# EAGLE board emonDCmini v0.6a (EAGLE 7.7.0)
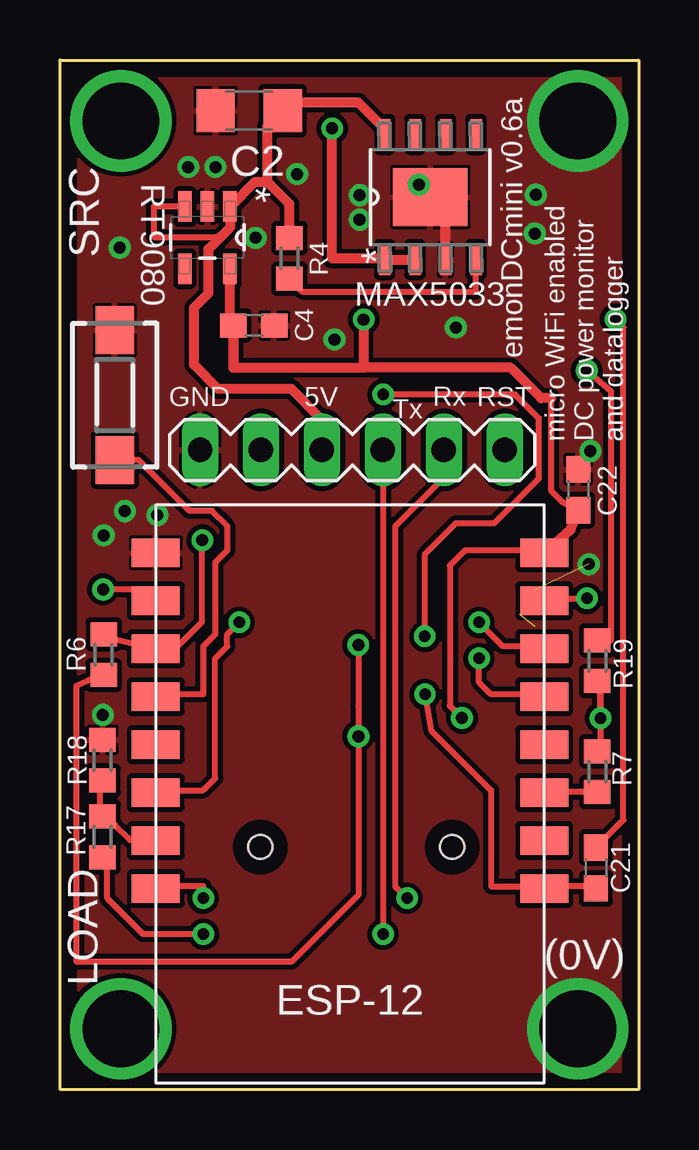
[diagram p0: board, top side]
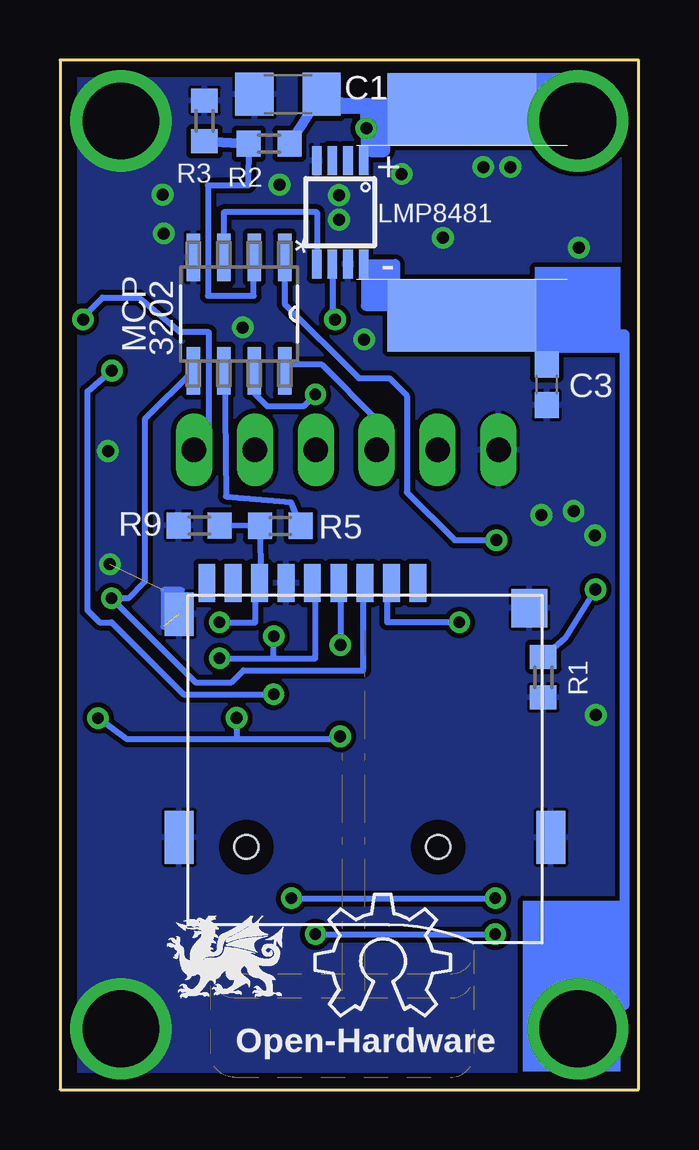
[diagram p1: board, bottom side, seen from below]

Size 24.13 x 42.93 mm. Coordinates in mm from the lower left corner, seen from the top.
Outline: 0,42.93 24.13,42.93 24.13,0 0,0 0,42.93
Copper layers (1*16): Top 0.035mm / dielectric 1.5mm / Bottom 0.035mm
Design rules "default *": minimum track width 10mil, minimum drill 19mil, track to track 8mil, track to pad 8mil, pad to pad 8mil, via to via 8mil, smd to smd 8mil, copper to edge 25mil, drill to drill 8mil, minimum pad ring 10mil, minimum via ring 8mil, stop-mask expansion 4mil, vias tented up to drill 0mil, thermal gap 5mil
Net classes: 1 power: width 1.016 mm; 2 thin_power: width 0.254 mm

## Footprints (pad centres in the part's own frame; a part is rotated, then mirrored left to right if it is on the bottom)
C1206 = smd 1.6 x 1.8: 1 -1.4,0; 2 1.4,0
C0603 = smd 1.1 x 1: 1 -0.85,0; 2 0.85,0
EBW_SERIES_10.5MM = smd 3 x 6.2: P$1 -4.3,0; P$2 4.3,0
ESP8266-ESP12 = smd 2 x 1.2: 1 16.2,2; 2 16.2,4; 3 16.2,6; 4 16.2,8; 5 16.2,10; 6 16.2,12; 7 16.2,14; 8 16.2,16; 9 0,16; 10 0,14; 11 0,12; 12 0,10; 13 0,8; 14 0,6; 15 0,4; 16 0,2
MA06-1 = drill 1.016 long: 1 0,0; 2 2.54,0; 3 5.08,0; 4 7.62,0; 5 10.16,0; 6 12.7,0
S-PDSO-G08 = smd 0.4 x 1.2: 1 -0.975,-2.157; 2 -0.325,-2.157; 3 0.325,-2.157; 4 0.975,-2.157; 5 0.975,2.157; 6 0.325,2.157; 7 -0.325,2.157; 8 -0.975,2.157
21-0111D_SBE-14-L = smd 1.295 x 0.483: 1 -2.603,1.905; 2 -2.603,0.635; 3 -2.603,-0.635; 4 -2.603,-1.905; 5 2.603,-1.905; 6 2.603,-0.635; 7 2.603,0.635; 8 2.603,1.905 | smd 2.413 x 3.099: EPAD 0,0
SOIC127P600X175-8N = smd 1.981 x 0.559: 1 -2.362,1.905; 2 -2.362,0.635; 3 -2.362,-0.635; 4 -2.362,-1.905; 5 2.362,-1.905; 6 2.362,-0.635; 7 2.362,0.635; 8 2.362,1.905
R0603 = smd 1 x 1.1: 1 -0.85,0; 2 0.85,0
TSOT-23-5 = smd 1.27 x 0.559: 1 -1.295,0.94; 2 -1.295,0; 3 -1.295,-0.94; 4 1.295,-0.94; 5 1.295,0.94
DTSM-3 = smd 2 x 1.6: 1 -2.7,0; 2 2.7,0
TF-MICRO-SD_PP3* = smd 0.7 x 1.6: 1 2.2,11; 2 1.1,11; 3 0,11; 4 -1.1,11; 5 -2.2,11; 6 -3.3,11; 7 -4.4,11; 8 -5.5,11; CD -6.6,11 | smd 1.2 x 2.2: MT1 -7.75,0.4; MT2 7.75,0.4 | smd 1.2 x 1.8: MT3 -7.75,9.7 | smd 1.5 x 1.6: MT4 6.85,9.95 | hole 1: -4.95,0; 3.05,0

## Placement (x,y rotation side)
C1  100V 47uF MLCC  [C1206]  14.62,41.5 180 bottom
C2  22uF 6.3V K7R MLCC  [C1206]  7.89,40.81 180 top
C3  0.1uF MLCC 100V  [C0603]  3.84,29.39 270 bottom
C4  1uF MLCC  [C0603]  8.09,31.86 0 top
C21  100nF 6V MLCC  [C0603]  22.35,9.25 90 top
C22  100nF 6V MLCC  [C0603]  21.61,25.01 270 top
EBW_SERIES_10.5  EBW_SERIES_10.5MM  [EBW_SERIES_10.5MM]  7.37,36.58 90 bottom
ESP-12  ESP8266_ESP-12  [ESP8266-ESP12]  20.19,24.38 180 top
FTDI1  FTDI-ESP  [MA06-1]  18.54,26.67 180 top
LMP8481  LMP8481-H  [S-PDSO-G08]  12.45,36.58 180 bottom
LOGO1  OSHW_LOGO_6MILX0200-NT  [OSHW_6X200_NOTEXT]  13.5,3.07 0 bottom
MAX5033  MAX5023TASA-T21-0111D_SBE-14-L  [21-0111D_SBE-14-L]  15.44,37.21 90 top
MCP3202  MCP3202-BI/SN  [SOIC127P600X175-8N]  16.66,32.33 270 bottom
R1  10k  [R0603]  3.98,17.2 270 bottom
R2  100K >70V  [R0603]  15.41,39.44 0 bottom
R3  5.9K  [R0603]  18.1,40.38 270 bottom
R4  10k  [R0603]  9.57,34.66 270 top
R5  10k  [R0603]  14.94,23.5 0 bottom
R6  10k  [R0603]  1.83,18.14 270 top
R7  10k  [R0603]  22.4,13.26 90 top
R9  6.98k  [R0603]  18.32,23.52 0 bottom
R17  5.6k  [R0603]  1.78,10.54 90 top
R18  10k  [R0603]  1.78,13.74 90 top
R19  10k  [R0603]  22.4,17.88 270 top
RT9080  RT9080-33GJ5  [TSOT-23-5]  6.15,35.52 270 top
S1  DTSM-3  [DTSM-3]  2.29,28.96 270 top
TFWF1-EBXX-1X0X  MICRO-SD3  [TF-MICRO-SD_PP3*]  11.41,10.12 0 bottom
U$3  [DRAGON_LOGO_NOTEXT]  17.07,5.51 0 bottom

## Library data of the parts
C1-C4 C21 C22 R1 R4 R6 R7 R17-R19 = rcl
EBW_SERIES_10.5 = EBW series shunt
ESP-12 = ESP8266-ESP12
FTDI1 = JeeLabs
LMP8481 = lmp8481b
LOGO1 = ohw-logo; OC_FARNELL: unknown
MAX5033 = MAX5053; MANUFACTURER_PART_NUMBER: max5033; VENDOR: MAXIM
MCP3202 = Microchip-MCP3202-BI_SN; MPN: MCP3202-BI/SN; OC_FARNELL: 1196803; OC_NEWARK: 96K3721; PACKAGE: SOIC-8; SUPPLIER: Microchip
R2 = rcl; MPN: MCWR06X1003FTL
R3 R5 R9 = rcl; MPN: MCWR06X5901FTL
RT9080 = TSOT-23-5 REGULATOR 3.3v; OC_FARNELL: 2679852; PACKAGE: SOT-23-5
S1 = switch-tact
TFWF1-EBXX-1X0X = TFWF1-EBXX-1X0X
U$3 = DRAGON_LOGO

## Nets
3.3V: C4.1 C22.2 ESP-12.16 LMP8481.6 R6.2 R7.2 R19.2 RT9080.5 TFWF1-EBXX-1X0X.4
+5V: C2.1 FTDI1.4 MAX5033.8 MCP3202.8 R4.1 RT9080.1 RT9080.3
ADC: ESP-12.10
ADC_CSENSE: LMP8481.5 MCP3202.3
ADC_VSENSE: MCP3202.2 R2.1 R3.2
CH_PD: ESP-12.11 R7.1
ESPRX: ESP-12.7 R17.2 R18.1
ESPTX: ESP-12.8 FTDI1.2
GND [thin_power]: C1.2 C2.2 C3.2 C4.2 C22.1 ESP-12.1 FTDI1.6 LMP8481.4 LMP8481.7 MAX5033.3 MAX5033.EPAD MCP3202.4 R1.2 R3.1 R9.1 R18.2 RT9080.2 S1.1 TFWF1-EBXX-1X0X.6 TFWF1-EBXX-1X0X.MT1 TFWF1-EBXX-1X0X.MT2 TFWF1-EBXX-1X0X.MT3 TFWF1-EBXX-1X0X.MT4
GPIO0: ESP-12.4 S1.2
GPIO2: ESP-12.3 MCP3202.1 R6.1
GPIO4: ESP-12.6 TFWF1-EBXX-1X0X.2
GPIO5: ESP-12.5
GPIO12: ESP-12.14 R5.1 R9.2 TFWF1-EBXX-1X0X.7
GPIO12A: MCP3202.6 R5.2
GPIO13: ESP-12.15 MCP3202.5 TFWF1-EBXX-1X0X.3
GPIO14: ESP-12.13 MCP3202.7 TFWF1-EBXX-1X0X.5
GPIO15: ESP-12.2 R1.1
LOAD- [power]: C3.1 EBW_SERIES_10.5.P$1 LMP8481.8
N$1: MAX5033.4 R4.2
N$36: FTDI1.3 R17.1
RESTESP: C21.1 ESP-12.9 R19.1
RST: C21.2 FTDI1.1
SOURCE+ [power]: C1.1 EBW_SERIES_10.5.P$2 LMP8481.1 MAX5033.1 MAX5033.2 R2.2

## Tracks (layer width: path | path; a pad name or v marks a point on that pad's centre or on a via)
3.3V  (via drill 0.48, 0.5)
  Top 0.254: R19.2 | 21.97,14.22 R7.2 22.54,14.19 22.54,16.73 R19.2 | R6.2 1.13,17.03 0.69,16.84 0.69,5.33 9.65,5.33 12.45,8.13 v12.45,14.73 12.44,16.01 v12.44,18.54 | C22.2 20.98,24.48 20.48,24.98 20.48,28.83 | v22.54,15.49 22.53,17.15 R19.2 | ESP-12.16 20.07,22.48 16.89,22.48 16.26,21.84 16.26,16 v16.76,15.49 v16.77,15.49
  Top 0.406: C22.2 21.29,23.35 ESP-12.16 | 12.66,30.1 18.8,30.1 20.07,28.82 20.48,28.83 | 7.24,30.11 | 7.24,30.11 C4.1 | C4.1 7.09,31.86 RT9080.5 | v12.66,32.11 12.66,30.1 | C4.1 7.24,30.1 12.66,30.1
  Bottom 0.254: LMP8481.6 12.77,32.22 | TFWF1-EBXX-1X0X.4 12.44,21.12 v12.44,18.54 | v22.54,15.49 21.34,14.61 16.76,14.61 | 16.76,14.61 12.45,14.61 v12.45,14.73 | v16.76,15.49 16.76,14.61
  Bottom 0.406: 12.77,32.22 v12.66,32.11
+5V
  Top 0.254: 6.69,35.54 6.69,35.55 3.91,35.55 3.91,36.82 RT9080.3
  Top 0.406: FTDI1.4 10.92,27.91 9.65,29.21 6.6,29.21 5.59,30.23 5.59,32.6 6.2,33.2 6.2,35.05 6.69,35.54 7.11,35.96 | 9.29,41.05 C2.1 | R4.1 9.57,36.92 8.64,37.85 | RT9080.1 7.11,36.82 8.14,37.85 8.64,37.85 | MAX5033.8 13.54,40.1 13.49,40.1 12.45,41.15 9.62,41.15 C2.1 | C2.1 8.64,40.16 8.64,37.85
  Top 0.424: 7.11,35.96 7.11,36.82
  Bottom 0.254: MCP3202.8 arc90 14.5,30.23 13.21,30.23 10.92,27.94 FTDI1.4
ADC_CSENSE
  Bottom 0.254: MCP3202.3 17.3,36.58 13.42,36.58 LMP8481.5
ADC_VSENSE
  Bottom 0.254: 16,34.7 MCP3202.2 16.05,34.7 16.05,33.1 17.96,33.1 17.96,37.69 16.29,37.69 R2.1
  Bottom 0.406: R3.2 R2.1
CH_PD
  Top 0.254: R7.1 20.32,12.41 ESP-12.11
ESPRX
  Top 0.254: 4.11,10.38 arc90 ESP-12.7 | 3.56,10.41 3.97,10.41 ESP-12.7 | 1.9,11.37 R17.2 | R18.1 1.75,12.79 1.68,12.48 1.68,11.37 1.75,11.37 R17.2 | 3.56,10.41 2.92,10.41 2.29,11.05 R17.2 | 3.56,10.41 ESP-12.7
ESPTX  (via drill 0.48)
  Top 0.254: v5.98,7.98 5.98,8.48 4.48,8.48 ESP-12.8 | v14.48,7.98 13.98,8.48 13.98,23.48 15.98,25.48 15.98,26.48 FTDI1.2
  Bottom 0.254: v14.48,7.98 v5.98,7.98
GND  (via drill 0.5, 3.2)  (2 unrouted)
  Top 0.254: ESP-12.1 4.19,22.48 4.22,22.29
  Top 0.406: MAX5033.3 16.08,36.58
  Bottom 0.254: 19.05,20.83 19.81,20.83 19.81,19.3
  other vias: 19.84,37.31 1.79,15.62 2.71,24.13 4.06,23.96 16.51,31.78 9.88,38.18 12.5,37.29 11.45,31.28 21.59,2.54 21.59,40.39 22.05,21.91 14.97,37.72 6.48,38.46 12.5,36.27 1.82,23.11 19.8,35.7 5.35,38.46 2.49,35.1 8.16,35.51 22.12,26.62
  pour Top: 0.25,42.67 23.88,42.67 23.88,0.25 0.25,0.25
  pour Bottom: 0.25,42.67 23.88,42.67 23.88,0.25 0.25,0.25
GPIO0
  Top 0.254: S1.2 3.28,26.26 5.4,24.13 6.35,24.13 6.96,23.52 6.98,23.48 6.98,22.48 6.48,21.98 6.48,18.98 5.98,18.48 5.98,16.48 4.48,16.48 ESP-12.4
GPIO2  (via drill 0.5)
  Top 0.254: R6.1 1.84,18.89 ESP-12.3 4.8,18.38 5.92,19.5 5.92,23.15 v5.93,22.91
  Bottom 0.254: MCP3202.1 14.76,32.75 11.67,29.66 10.39,29.66 9.66,28.94 9.66,24.91 7.67,22.91 v5.93,22.91
GPIO4  (via drill 0.48)
  Top 0.254: v7.48,19.48 6.98,18.98 6.98,18.48 6.48,17.98 6.48,12.98 5.98,12.48 4.48,12.48 ESP-12.6
  Bottom 0.254: v7.48,19.48 10.48,19.48 10.48,20.98 TFWF1-EBXX-1X0X.2
GPIO12  (via drill 0.48)
  Top 0.254: v17.48,19.48 18.48,18.48 19.98,18.48 ESP-12.14
  Bottom 0.254: v17.48,19.48 15.98,19.48 15.98,20.98 TFWF1-EBXX-1X0X.7 15.98,21.42 15.77,21.25 R5.1 R9.2
GPIO12A
  Bottom 0.254: MCP3202.6 17.27,29.97 17.21,24.74 14.52,24.5 R5.2
GPIO13  (via drill 0.48)
  Top 0.254: v21.98,20.48 20.48,20.48 ESP-12.15
  Bottom 0.254: TFWF1-EBXX-1X0X.3 11.48,20.98 11.48,17.48 16.48,17.48 16.98,16.98 18.48,16.98 v21.98,20.48 21.27,20.48 20.59,21.17 20.59,27.95 MCP3202.5
GPIO14  (via drill 0.48)
  Top 0.254: v17.48,17.98 17.48,16.98 17.98,16.48 19.98,16.48 ESP-12.13 | v13.48,28.98 18.98,28.98 19.98,27.98 19.98,25.48 18.11,23.62 16.51,23.62 15.22,22.33 v15.21,18.9
  Bottom 0.254: v17.48,17.98 15.22,17.98 | 15.22,17.98 13.48,17.98 13.48,20.98 TFWF1-EBXX-1X0X.5 | v13.48,28.98 13.98,28.48 15.48,28.48 15.98,28.98 15.98,29.48 MCP3202.7 | 15.22,17.98 v15.21,18.9
GPIO15  (via drill 0.5)
  Top 0.254: ESP-12.2 3.52,20.85 v1.8,20.85
  Bottom 0.254: v1.8,20.85 3.09,18.81 R1.1
LOAD-  (via drill 3.2)
  Bottom 0.254: 11.43,34.29 11.47,34.33 LMP8481.8
  Bottom 0.406: 1.2,31.5 6.59,31.5 EBW_SERIES_10.5.P$1 7.37,33.27 10.16,33.27 10.16,34.42 LMP8481.8 | 1.2,31.5 0.58,31.5 0.58,3.53 2.54,3.53 v2.54,2.54 | 11.43,34.29 11.37,34.31 11.37,32.67 10.28,32.65 10.28,32.66 10.34,32.66 10.34,34.17 11.19,34.17 11.19,34.18 11.18,34.18 11.18,32.99 10.55,32.99 10.55,32.94 10.59,32.94 10.59,33.92 10.87,33.92 10.87,33.96 10.89,33.96 10.89,33.23 | C3.1 3.49,31.64 1.2,31.5
N$1
  Top 0.254: R4.2 10.1,33.27 17.35,33.27 MAX5033.4
N$36  (via drill 0.48)
  Top 0.254: v5.98,6.48 3.48,6.48 1.98,7.98 1.98,9.48 R17.1 | v13.48,6.48 13.48,26.48 FTDI1.3
  Bottom 0.254: v13.48,6.48 v5.98,6.48
RESTESP  (via drill 0.48, 0.5)
  Top 0.254: C21.1 21.97,8.51 20.7,8.51 ESP-12.9 19.98,8.48 17.98,8.48 17.98,12.48 15.48,14.98 v15.22,16.48 | R19.1 22.99,18.73 22.99,29.1 v21.97,29.98
  Bottom 0.254: v15.22,16.48 18.98,16.48 21.98,19.48 22.48,19.48 22.98,19.98 22.98,29.11 v21.97,29.98
RST  (via drill 0.5)
  Top 0.254: C21.2 23.49,11.24 23.49,31.78 v23.17,32.11
  Bottom 0.254: v23.17,32.11 23.17,32.2 22.35,33.02 20.83,33.02 19.13,31.57 17.93,31.57 17.93,26.67 FTDI1.1
SOURCE+  (via drill 0.5, 3.2)
  Top 0.406: MAX5033.1 | v11.35,40.07 11.35,34.65 13.54,34.65 MAX5033.1 | MAX5033.1 MAX5033.2
  Bottom 0.254: v11.35,40.07 11.47,40.12 | 11.47,40.12 LMP8481.1 | 11.49,40.85 11.49,40.02 | 11.49,40.02 11.49,39.94 11.43,39.88 | 11.2,40.99 11.34,40.85 11.49,40.85 | 11.49,40.87 11.49,40.85 | 11.47,40.12 11.49,40.02
  Bottom 0.406: 7.37,41.63 EBW_SERIES_10.5.P$2 7.37,39.62 10.66,39.62 10.66,39.63 | 2.29,40.89 2.54,40.89 v2.54,40.39 | R2.2 C1.1 11.49,40.85 | 10.16,41.15 12.7,41.15 12.7,40.89 10.67,40.89 10.66,41.02
  Bottom 0.61: 10.66,41.02 10.66,39.63 10.67,39.16 11.1,39.16 11.1,40.89 11.2,40.99
  Bottom 1.016: 2.29,40.89 7.37,40.89 EBW_SERIES_10.5.P$2
(copper drawn outside any net)
  shapes: Bottom area x3

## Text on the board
bPlace: Open-Hardware
tNames: SRC | emonDCmini v0.6a | GND | 5V | Rx | RST | Tx | micro WiFi enabled / DC power monitor / and datalogger | LOAD | (0V)
bNames: 3202 | MCP
_tsilk: Designed in | North Wales | Made in UK
_bsilk: SMT V0.6 rev3 | emonTx | wireless energy monitoring node | SMT V0.6 rev3 | emonTx | SMT V0.6 rev3 | emonTx | Technology that helps us live within ecological limits | wireless energy monitoring node | wireless energy monitoring node | Designed in North Wales UK by Glyn Hudson & Trystan Lea | Technology that helps us live within ecological limits | Technology that helps us live within ecological limits | Designed in North Wales UK by Glyn Hudson & Trystan Lea | 165mm ant | 433Mhz | Designed in North Wales UK by Glyn Hudson & Trystan Lea | 165mm ant | 165mm ant | 433Mhz | 433Mhz | 868Mhz | 82mm ant | 82mm ant | 82mm ant | 868Mhz | 868Mhz | 78mm ant | 915Mhz | 78mm ant | 915Mhz | 78mm ant | 915Mhz | 165mm ant | 433Mhz | 82mm ant | 868Mhz | 78mm ant | 915Mhz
